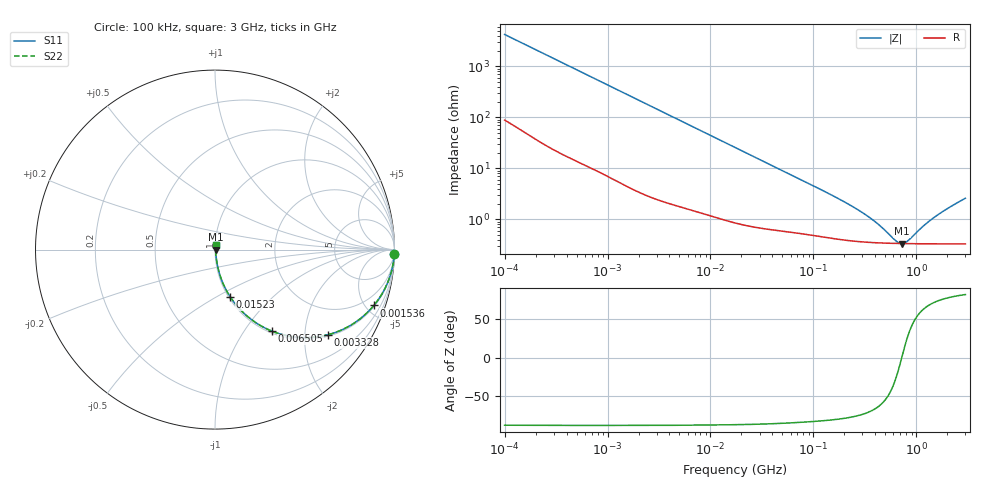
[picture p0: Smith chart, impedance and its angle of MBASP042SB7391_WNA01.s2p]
! MBASP042SB7391_WNA01  S-PARAMETER MODEL  ( Standard Model )
! Model Generated by TAIYO YUDEN Corporation (https://www.yuden.co.jp/en/)
! Version 1.0
! TAIYO YUDEN Control No. 250312
! Copyright(c) 2025 TAIYO YUDEN CO.,LTD. All Rights Reserved.
! Product Description (link to TY-COMPAS)
! https://ds.yuden.co.jp/TYCOMPAS/or/detail?pn=MBASP042SB7391KWNA01&u=M
! Products Name : Multilayer Ceramic Capacitors
! Characteristics :
!  Capacitance : 390 [pF] , Rated Voltage : 2.5 [V] , TCC : X7R
!  Case Size : 0.4 x 0.2 / 0.016 x 0.008 [mm/inch] , Thickness : 0.2 / 0.008 [mm/inch]
!  (Conditions: Temperature = 25 [degC] , DC Bias Voltage = 0 [V])
! External Node Assignments :
!  1  o---| |---o  2
! GND o---------o GND
! Frequency Range : 100kHz  -  3GHz  [ 401 STEP ]
# MHZ S RI R 50
! Freq[MHz].  S11 Real  S11 Imag  S21 Real  S21 Imag  S12 Real  S12 Imag  S22 Real  S22 Imag
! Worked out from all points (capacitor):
!   401 points, 100 kHz to 3 GHz, reference 50 ohm
!   read as one part in series: C = 376 pF near 105.3 kHz
!   lowest |Z| = 333 mohm at 727 MHz (marker M1)
!   series resonance near 722.6 MHz, so ESL is about 130 pH
!   S11 on the Smith chart (normalised r, x): 100 kHz: 3, -84; 1.536 MHz: 1.09, -5.65; 3.328 MHz: 1.05, -2.62; 6.505 MHz: 1.03, -1.35; 15.23 MHz: 1.02, -0.58; 3 GHz: 1.01, +0.05
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0.1  0.9989 -0.0236  0.00105 0.0236  0.00105 0.0236  0.9989 -0.0236
0.562235  0.9812 -0.1281  0.0188 0.1281  0.0188 0.1281  0.9812 -0.1281
1.536162  0.8849 -0.3114  0.1151 0.3114  0.1151 0.3114  0.8849 -0.3114
2.203618  0.7922 -0.3979  0.2078 0.3979  0.2078 0.3979  0.7922 -0.3979
3.161081  0.6533 -0.4675  0.3467 0.4675  0.3467 0.4675  0.6533 -0.4675
3.328291  0.6301 -0.4742  0.3699 0.4742  0.3699 0.4742  0.6301 -0.4742
4.652942  0.47 -0.4894  0.53 0.4894  0.53 0.4894  0.47 -0.4894
6.504802  0.3169 -0.4542  0.6831 0.4542  0.6831 0.4542  0.3169 -0.4542
9.824692  0.1743 -0.3665  0.8257 0.3665  0.8257 0.3665  0.1743 -0.3665
15.22638  0.0852 -0.264  0.9148 0.264  0.9148 0.264  0.0852 -0.264
17.7727  0.0656 -0.2315  0.9344 0.2315  0.9344 0.2315  0.0656 -0.2315
38.50681  0.0193 -0.1131  0.9807 0.1131  0.9807 0.1131  0.0193 -0.1131
97.38194  0.00691 -0.0456  0.9931 0.0456  0.9931 0.0456  0.00691 -0.0456
287.4592  0.00379 -0.0137  0.9962 0.0137  0.9962 0.0137  0.00379 -0.0137
401.8672  0.00351 -0.00805  0.9965 0.00805  0.9965 0.00805  0.00351 -0.00805
547.5153  0.00338 -0.00365  0.9966 0.00365  0.9966 0.00365  0.00338 -0.00365
655.7614  0.00333 -0.00126  0.9967 0.00126  0.9967 0.00126  0.00333 -0.00126
726.971  0.00332 7.99e-05  0.9967 -7.99e-05  0.9967 -7.99e-05  0.00332 7.99e-05
826.9535  0.00331 0.00176  0.9967 -0.00176  0.9967 -0.00176  0.00331 0.00176
1186.261  0.00333 0.00672  0.9967 -0.00672  0.9967 -0.00672  0.00333 0.00672
1575.075  0.0034 0.0112  0.9966 -0.0112  0.9966 -0.0112  0.0034 0.0112
3000  0.00391 0.0255  0.9961 -0.0255  0.9961 -0.0255  0.00391 0.0255
